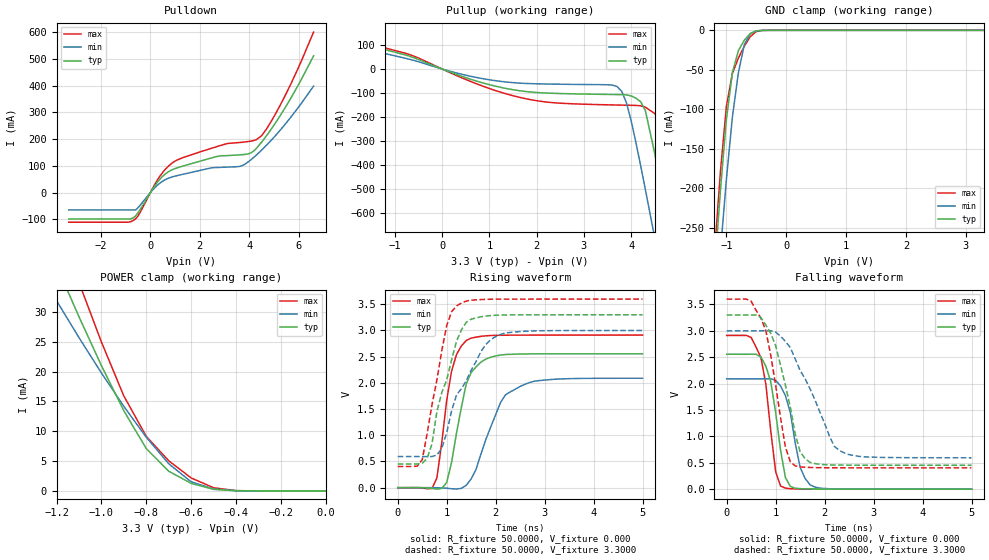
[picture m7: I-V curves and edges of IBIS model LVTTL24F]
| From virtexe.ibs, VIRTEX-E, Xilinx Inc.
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|   Model LVTTL24F
[Model]   LVTTL24F
Model_type   I/O
Polarity   Non-Inverting
Enable   Active-Low
Vinl =   0.800V
Vinh =   2.000V
Vmeas =   1.4000V
Cref =  35.0000pF
Rref =   1.0000M
Vref =  0.000V
C_comp   5.0000pF   4.0000pF   6.0000pF
[Temperature Range]   25.0000   100.0000   0.000
[Voltage Range]   3.3000V   3.0000V   3.6000V
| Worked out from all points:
|   slope of the pulldown table from 0 to 0.495 V, typ, clamps not added: 8.13 ohm
|   slope of the pullup table from 0 to 0.495 V, typ, clamps not added: 13.9 ohm
|   GND clamp passes 1 mA (typ) near -0.51 V on its own axis
|   POWER clamp passes 1 mA (typ) near -0.57 V on its own axis
|   rising waveform, R_fixture 50.0000, V_fixture 0.000: 20-80 % time 323ps typ, 508ps min, 275ps max; typ from 0 V to 2.56 V
|   rising waveform, R_fixture 50.0000, V_fixture 3.3000: 20-80 % time 453ps typ, 651ps min, 369ps max; typ from 0.452 V to 3.3 V
|   falling waveform, R_fixture 50.0000, V_fixture 0.000: 20-80 % time 246ps typ, 268ps min, 236ps max; typ from 2.56 V to 0 V
|   falling waveform, R_fixture 50.0000, V_fixture 3.3000: 20-80 % time 412ps typ, 694ps min, 347ps max; typ from 3.3 V to 0.452 V
[Pulldown]
| voltage   I(typ)   I(min)   I(max)
-3.3V     -98.33mA   -65mA      -110.7mA
-800mV    -98.33mA   -65mA      -109.1mA
-500mV    -75.76mA   -56.49mA   -87.36mA
400mV     51.81mA    36.52mA    63.47mA
900mV     86.5mA     59.29mA    112.3mA
2.7V      135.6mA    94.02mA    172.5mA
3.7V      142mA      100.7mA    188.5mA
4.1V      150.7mA    125.7mA    193.3mA
4.5V      189.1mA    159.2mA    213.1mA
4.9V      239.3mA    197.3mA    268.9mA
5.5V      325.6mA    261.6mA    372.6mA
6.6V      512mA      398.9mA    601mA
[Pullup]
| voltage   I(typ)   I(min)   I(max)
-3.3V     164mA      145.7mA    167.3mA
-800mV    59.77mA    45.78mA    67.04mA
1.3V      -78.71mA   -52.7mA    -99.97mA
3.7V      -106.1mA   -72.4mA    -149.7mA
3.9V      -107.5mA   -140.1mA   -150.5mA
4.2V      -135.5mA   -401.1mA   -152.8mA
4.3V      -172.4mA   -500.5mA   -158.4mA
4.5V      -352mA     -704.4mA   -185.3mA
4.7V      -569.5mA   -912.2mA   -261.9mA
4.9V      -796mA     -1.122A    -460.6mA
5.1V      -1.026A    -1.333A    -688.6mA
6.6V      -2.792A    -2.941A    -2.5A
[GND_clamp]
| voltage   I(typ)   I(min)   I(max)
-3.3V     -2.749A    -2.594A    -2.805A
-1.2V     -306mA     -377.1mA   -282.7mA
-1.1V     -202.5mA   -280mA     -178.8mA
-1V       -112.5mA   -188.5mA   -95.98mA
-900mV    -53.5mA    -109.7mA   -54.53mA
-800mV    -25.67mA   -53.59mA   -35.13mA
-700mV    -12.44mA   -17.88mA   -19.82mA
-600mV    -3.982mA   -4.202mA   -7.865mA
-500mV    -601.5uA   -800.3uA   -1.508mA
-400mV    -51.05uA   -119.3uA   -124.3uA
3.3V      18.74nA    3.634uA    18.92nA
[POWER_clamp]
| voltage   I(typ)   I(min)   I(max)
-3.3V     237mA      175.9mA    284.4mA
-1.3V     46.69mA    38.29mA    56.33mA
-1.2V     37.79mA    31.9mA     45.45mA
-1.1V     29.2mA     25.71mA    34.95mA
-1V       21.01mA    19.78mA    24.97mA
-900mV    13.43mA    14.17mA    15.91mA
-800mV    7.091mA    8.993mA    9.139mA
-700mV    3.305mA    4.554mA    5.052mA
-600mV    1.265mA    1.529mA    2.172mA
-500mV    263.8uA    333.6uA    531.5uA
-400mV    22.63uA    44.12uA    49.77uA
0V        18.8nA     38.36nA    22.53nA
[Ramp]
| variable   typ   min   max
dV/dt_r   1.5330/0.3406n   1.2534/0.5304n   1.7472/0.2600n
dV/dt_f   1.7086/0.4323n   1.4433/0.6840n   1.9178/0.3388n
R_load = 50.0000
[Rising Waveform]
R_fixture = 50.0000
V_fixture = 0.000
| time   V(typ)   V(min)   V(max)
0s        1.342uV    1.532uV    1.321uV
700ps     -12.7mV    572.7uV    -15.4mV
800ps     -28.59mV   -1.877mV   186.3mV
1ns       98.02mV    -10.74mV   1.666V
1.2ns     1.038V     -25.72mV   2.541V
1.4ns     1.983V     46.12mV    2.81V
1.7ns     2.396V     646.4mV    2.889V
2.1ns     2.531V     1.626V     2.909V
2.3ns     2.545V     1.829V     2.911V
5ns       2.555V     2.089V     2.912V
[Rising Waveform]
R_fixture = 50.0000
V_fixture = 3.3000
V_fixture_min = 3.0000
V_fixture_max = 3.6000
| time   V(typ)   V(min)   V(max)
0s        452.1mV    593.7mV    403.5mV
500ps     467.3mV    594mV      534.2mV
700ps     838.2mV    594.2mV    1.583V
900ps     1.815V     749.8mV    2.616V
1ns       2.057V     1.047V     3.093V
1.2ns     2.792V     1.77V      3.469V
1.5ns     3.216V     2.242V     3.578V
1.8ns     3.276V     2.734V     3.595V
2.1ns     3.294V     2.926V     3.599V
5ns       3.3V       3V         3.6V
[Falling Waveform]
R_fixture = 50.0000
V_fixture = 0.000
| time   V(typ)   V(min)   V(max)
0s        2.555V     2.089V     2.912V
500ps     2.557V     2.089V     2.873V
700ps     2.503V     2.089V     2.49V
900ps     2.037V     2.091V     1.103V
1ns       1.453V     2.062V     332.8mV
1.1ns     739.3mV    1.955V     58.62mV
1.3ns     53.4mV     1.45V      8.987mV
1.5ns     9.431mV    415.2mV    3.395mV
1.7ns     4.681mV    83.88mV    2.031mV
5ns       72.92uV    310.5uV    58.06uV
[Falling Waveform]
R_fixture = 50.0000
V_fixture = 3.3000
V_fixture_min = 3.0000
V_fixture_max = 3.6000
| time   V(typ)   V(min)   V(max)
0s        3.3V       3V         3.6V
500ps     3.3V       3V         3.56V
700ps     3.249V     3V         3.238V
900ps     2.95V      3.001V     2.535V
1.2ns     1.966V     2.798V     793.7mV
1.4ns     1.042V     2.466V     441.1mV
1.5ns     709.2mV    2.248V     421.8mV
1.7ns     507.7mV    1.904V     411.2mV
2.3ns     456.3mV    736mV      404.7mV
5ns       452.3mV    594.5mV    403.7mV
